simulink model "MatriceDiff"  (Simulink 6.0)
settings: Solver=ode45  StartTime=0  StopTime=17*t0  RelTol=1e-3
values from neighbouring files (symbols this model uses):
  b = S/Sm    (= 0.1)    [Constantes.m]    (also in ConstantesBck.m)
  beta = 0.95    [Constantes.m]    (also in ConstantesBck.m; ResCourV1.m = 1; ResCrV1.m = 1; ResEnerV1.m = 1)
  C = 1    [Constantes.m]    (also in ConstantesBck.m)
  gk = 36    [Constantes.m]    (also in ConstantesBck.m; sim_hh.m)
  gl = 0.3    [Constantes.m]    (also in ConstantesBck.m; sim_hh.m)
  gna = 120    [Constantes.m]    (also in ConstantesBck.m; sim_hh.m)
  h0 = 0.5961    [Constantes.m]    (also in ConstantesBck.m)
  m0 = 0.0529    [Constantes.m]    (also in ConstantesBck.m)
  mK = 0    [Constantes.m]    (also in ConstantesBck.m)
  mL = 0    [Constantes.m]    (also in ConstantesBck.m)
  mNa = 0    [Constantes.m]    (also in ConstantesBck.m)
  N = [6,8,5,5,7,1,2,6,9,1,1,9,4,8,8,7]    [Constantes.m]    (also in ConstantesBck.m; ImpedanceZtissus.m = 100; Ztissus.m = 100; charge.m = N(:,2))
  n0 = 0.3177    [Constantes.m]    (also in ConstantesBck.m)
  rapportIE = 10    [Constantes.m]
  Sm = 3.14e-2    (= 0.0314)    [Constantes.m]    (also in ConstantesBck.m = 0.000314)
  t0 = 2E-3    (= 0.002)    [Constantes.m]    (also in ConstantesBck.m = 0.001)
  Vk = -82    [Constantes.m]    (also in ConstantesBck.m)
  Vl = -59    [Constantes.m]    (also in ConstantesBck.m)
  Vna = 45    [Constantes.m]    (also in ConstantesBck.m)
  Vr = -70    [Constantes.m]    (also in ConstantesBck.m)
undefined symbols (not defined in the file or in its folder): ln
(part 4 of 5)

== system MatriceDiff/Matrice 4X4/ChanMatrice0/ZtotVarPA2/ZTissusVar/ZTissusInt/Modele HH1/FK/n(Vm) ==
  note: V
  note: alpha_*(1-n)
  note: beta_n*n
  note: n
  note: n
  Vm : Inport  Port=1  LatchInput=off
  (1-n) : Fcn  Expr=1-u
  Integrator1 : Integrator  InitialCondition=n0
  Product : Product
  Product1 : Product
  Sum1 : Sum  Inputs=+-
  V : Fcn  Expr=u-Vr
  alpha_n : Fcn  Expr=(0.01*(10-u))/(exp((10-u)/10)-1)
  beta_n : Fcn  Expr=0.125*exp(-u/80)
  n : Outport  InitialOutput=0
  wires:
  V/1 -> alpha_n/1, beta_n/1
  alpha_n/1 -> Product/2
  (1-n)/1 -> Product/1
  beta_n/1 -> Product1/1
  Product/1 -> Sum1/1
  Product1/1 -> Sum1/2
  Sum1/1 -> Integrator1/1
  Integrator1/1 -> (1-n)/1, Product1/2, n/1
  Vm/1 -> V/1

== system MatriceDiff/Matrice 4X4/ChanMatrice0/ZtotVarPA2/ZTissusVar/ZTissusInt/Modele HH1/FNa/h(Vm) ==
  note: h
  note: h
  note: beta_h*h
  note: alpha_h*(1-h)
  note: V
  Vm : Inport  Port=1  LatchInput=off
  (1-h) : Fcn  Expr=1-u
  Integrator1 : Integrator  InitialCondition=h0
  Product : Product
  Product1 : Product
  Sum1 : Sum  Inputs=+-
  V : Fcn  Expr=u-Vr
  alpha_h : Fcn  Expr=0.07*exp(-u/20)
  beta_h : Fcn  Expr=1/(exp((30-u)/10)+1)
  h : Outport  InitialOutput=0
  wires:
  Vm/1 -> V/1
  Integrator1/1 -> h/1, Product1/2, (1-h)/1
  Sum1/1 -> Integrator1/1
  Product1/1 -> Sum1/2
  Product/1 -> Sum1/1
  beta_h/1 -> Product1/1
  (1-h)/1 -> Product/1
  alpha_h/1 -> Product/2
  V/1 -> beta_h/1, alpha_h/1

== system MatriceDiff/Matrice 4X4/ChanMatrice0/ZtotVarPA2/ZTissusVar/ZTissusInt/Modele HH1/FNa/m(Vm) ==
  note: m
  note: m
  note: beta_m*m
  note: alpha_m*(1-m)
  note: V
  Vm : Inport  Port=1  LatchInput=off
  (1-m) : Fcn  Expr=1-u
  Integrator1 : Integrator  InitialCondition=m0
  Product : Product
  Product1 : Product
  Sum1 : Sum  Inputs=+-
  V : Fcn  Expr=u-Vr
  alpha_m : Fcn  Expr=(0.1*(25-u))/(exp((25-u)/10)-1)
  beta_m : Fcn  Expr=4*exp(-u/18)
  n : Outport  InitialOutput=0
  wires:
  Vm/1 -> V/1
  Integrator1/1 -> n/1, Product1/2, (1-m)/1
  Sum1/1 -> Integrator1/1
  Product1/1 -> Sum1/2
  Product/1 -> Sum1/1
  beta_m/1 -> Product1/1
  (1-m)/1 -> Product/1
  alpha_m/1 -> Product/2
  V/1 -> beta_m/1, alpha_m/1

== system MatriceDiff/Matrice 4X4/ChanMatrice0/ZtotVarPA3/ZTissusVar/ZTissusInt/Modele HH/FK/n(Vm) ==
  note: V
  note: alpha_*(1-n)
  note: beta_n*n
  note: n
  note: n
  Vm : Inport  Port=1  LatchInput=off
  (1-n) : Fcn  Expr=1-u
  Integrator1 : Integrator  InitialCondition=n0
  Product : Product
  Product1 : Product
  Sum1 : Sum  Inputs=+-
  V : Fcn  Expr=u-Vr
  alpha_n : Fcn  Expr=(0.01*(10-u))/(exp((10-u)/10)-1)
  beta_n : Fcn  Expr=0.125*exp(-u/80)
  n : Outport  InitialOutput=0
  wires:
  V/1 -> alpha_n/1, beta_n/1
  alpha_n/1 -> Product/2
  (1-n)/1 -> Product/1
  beta_n/1 -> Product1/1
  Product/1 -> Sum1/1
  Product1/1 -> Sum1/2
  Sum1/1 -> Integrator1/1
  Integrator1/1 -> (1-n)/1, Product1/2, n/1
  Vm/1 -> V/1

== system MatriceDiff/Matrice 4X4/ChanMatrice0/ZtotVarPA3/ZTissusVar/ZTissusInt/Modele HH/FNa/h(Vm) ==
  note: h
  note: h
  note: beta_h*h
  note: alpha_h*(1-h)
  note: V
  Vm : Inport  Port=1  LatchInput=off
  (1-h) : Fcn  Expr=1-u
  Integrator1 : Integrator  InitialCondition=h0
  Product : Product
  Product1 : Product
  Sum1 : Sum  Inputs=+-
  V : Fcn  Expr=u-Vr
  alpha_h : Fcn  Expr=0.07*exp(-u/20)
  beta_h : Fcn  Expr=1/(exp((30-u)/10)+1)
  h : Outport  InitialOutput=0
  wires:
  Vm/1 -> V/1
  Integrator1/1 -> h/1, Product1/2, (1-h)/1
  Sum1/1 -> Integrator1/1
  Product1/1 -> Sum1/2
  Product/1 -> Sum1/1
  beta_h/1 -> Product1/1
  (1-h)/1 -> Product/1
  alpha_h/1 -> Product/2
  V/1 -> beta_h/1, alpha_h/1

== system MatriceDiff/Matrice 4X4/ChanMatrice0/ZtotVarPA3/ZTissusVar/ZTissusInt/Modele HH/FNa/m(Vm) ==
  note: m
  note: m
  note: beta_m*m
  note: alpha_m*(1-m)
  note: V
  Vm : Inport  Port=1  LatchInput=off
  (1-m) : Fcn  Expr=1-u
  Integrator1 : Integrator  InitialCondition=m0
  Product : Product
  Product1 : Product
  Sum1 : Sum  Inputs=+-
  V : Fcn  Expr=u-Vr
  alpha_m : Fcn  Expr=(0.1*(25-u))/(exp((25-u)/10)-1)
  beta_m : Fcn  Expr=4*exp(-u/18)
  n : Outport  InitialOutput=0
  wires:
  Vm/1 -> V/1
  Integrator1/1 -> n/1, Product1/2, (1-m)/1
  Sum1/1 -> Integrator1/1
  Product1/1 -> Sum1/2
  Product/1 -> Sum1/1
  beta_m/1 -> Product1/1
  (1-m)/1 -> Product/1
  alpha_m/1 -> Product/2
  V/1 -> beta_m/1, alpha_m/1

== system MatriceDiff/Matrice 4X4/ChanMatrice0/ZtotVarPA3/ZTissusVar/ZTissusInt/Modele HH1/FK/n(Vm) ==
  note: V
  note: alpha_*(1-n)
  note: beta_n*n
  note: n
  note: n
  Vm : Inport  Port=1  LatchInput=off
  (1-n) : Fcn  Expr=1-u
  Integrator1 : Integrator  InitialCondition=n0
  Product : Product
  Product1 : Product
  Sum1 : Sum  Inputs=+-
  V : Fcn  Expr=u-Vr
  alpha_n : Fcn  Expr=(0.01*(10-u))/(exp((10-u)/10)-1)
  beta_n : Fcn  Expr=0.125*exp(-u/80)
  n : Outport  InitialOutput=0
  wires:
  V/1 -> alpha_n/1, beta_n/1
  alpha_n/1 -> Product/2
  (1-n)/1 -> Product/1
  beta_n/1 -> Product1/1
  Product/1 -> Sum1/1
  Product1/1 -> Sum1/2
  Sum1/1 -> Integrator1/1
  Integrator1/1 -> (1-n)/1, Product1/2, n/1
  Vm/1 -> V/1

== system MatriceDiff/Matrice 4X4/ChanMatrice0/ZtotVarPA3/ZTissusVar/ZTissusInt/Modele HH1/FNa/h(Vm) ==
  note: h
  note: h
  note: beta_h*h
  note: alpha_h*(1-h)
  note: V
  Vm : Inport  Port=1  LatchInput=off
  (1-h) : Fcn  Expr=1-u
  Integrator1 : Integrator  InitialCondition=h0
  Product : Product
  Product1 : Product
  Sum1 : Sum  Inputs=+-
  V : Fcn  Expr=u-Vr
  alpha_h : Fcn  Expr=0.07*exp(-u/20)
  beta_h : Fcn  Expr=1/(exp((30-u)/10)+1)
  h : Outport  InitialOutput=0
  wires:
  Vm/1 -> V/1
  Integrator1/1 -> h/1, Product1/2, (1-h)/1
  Sum1/1 -> Integrator1/1
  Product1/1 -> Sum1/2
  Product/1 -> Sum1/1
  beta_h/1 -> Product1/1
  (1-h)/1 -> Product/1
  alpha_h/1 -> Product/2
  V/1 -> beta_h/1, alpha_h/1

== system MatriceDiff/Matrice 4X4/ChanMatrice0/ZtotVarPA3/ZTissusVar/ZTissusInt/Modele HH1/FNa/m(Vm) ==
  note: m
  note: m
  note: beta_m*m
  note: alpha_m*(1-m)
  note: V
  Vm : Inport  Port=1  LatchInput=off
  (1-m) : Fcn  Expr=1-u
  Integrator1 : Integrator  InitialCondition=m0
  Product : Product
  Product1 : Product
  Sum1 : Sum  Inputs=+-
  V : Fcn  Expr=u-Vr
  alpha_m : Fcn  Expr=(0.1*(25-u))/(exp((25-u)/10)-1)
  beta_m : Fcn  Expr=4*exp(-u/18)
  n : Outport  InitialOutput=0
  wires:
  Vm/1 -> V/1
  Integrator1/1 -> n/1, Product1/2, (1-m)/1
  Sum1/1 -> Integrator1/1
  Product1/1 -> Sum1/2
  Product/1 -> Sum1/1
  beta_m/1 -> Product1/1
  (1-m)/1 -> Product/1
  alpha_m/1 -> Product/2
  V/1 -> beta_m/1, alpha_m/1

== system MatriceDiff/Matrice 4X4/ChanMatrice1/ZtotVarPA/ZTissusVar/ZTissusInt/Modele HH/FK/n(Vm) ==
  note: V
  note: alpha_*(1-n)
  note: beta_n*n
  note: n
  note: n
  Vm : Inport  Port=1  LatchInput=off
  (1-n) : Fcn  Expr=1-u
  Integrator1 : Integrator  InitialCondition=n0
  Product : Product
  Product1 : Product
  Sum1 : Sum  Inputs=+-
  V : Fcn  Expr=u-Vr
  alpha_n : Fcn  Expr=(0.01*(10-u))/(exp((10-u)/10)-1)
  beta_n : Fcn  Expr=0.125*exp(-u/80)
  n : Outport  InitialOutput=0
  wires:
  V/1 -> alpha_n/1, beta_n/1
  alpha_n/1 -> Product/2
  (1-n)/1 -> Product/1
  beta_n/1 -> Product1/1
  Product/1 -> Sum1/1
  Product1/1 -> Sum1/2
  Sum1/1 -> Integrator1/1
  Integrator1/1 -> (1-n)/1, Product1/2, n/1
  Vm/1 -> V/1

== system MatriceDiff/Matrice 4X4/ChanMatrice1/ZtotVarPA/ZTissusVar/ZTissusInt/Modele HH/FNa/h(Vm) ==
  note: h
  note: h
  note: beta_h*h
  note: alpha_h*(1-h)
  note: V
  Vm : Inport  Port=1  LatchInput=off
  (1-h) : Fcn  Expr=1-u
  Integrator1 : Integrator  InitialCondition=h0
  Product : Product
  Product1 : Product
  Sum1 : Sum  Inputs=+-
  V : Fcn  Expr=u-Vr
  alpha_h : Fcn  Expr=0.07*exp(-u/20)
  beta_h : Fcn  Expr=1/(exp((30-u)/10)+1)
  h : Outport  InitialOutput=0
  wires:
  Vm/1 -> V/1
  Integrator1/1 -> h/1, Product1/2, (1-h)/1
  Sum1/1 -> Integrator1/1
  Product1/1 -> Sum1/2
  Product/1 -> Sum1/1
  beta_h/1 -> Product1/1
  (1-h)/1 -> Product/1
  alpha_h/1 -> Product/2
  V/1 -> beta_h/1, alpha_h/1

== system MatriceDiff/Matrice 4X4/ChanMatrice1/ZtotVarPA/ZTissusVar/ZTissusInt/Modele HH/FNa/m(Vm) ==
  note: m
  note: m
  note: beta_m*m
  note: alpha_m*(1-m)
  note: V
  Vm : Inport  Port=1  LatchInput=off
  (1-m) : Fcn  Expr=1-u
  Integrator1 : Integrator  InitialCondition=m0
  Product : Product
  Product1 : Product
  Sum1 : Sum  Inputs=+-
  V : Fcn  Expr=u-Vr
  alpha_m : Fcn  Expr=(0.1*(25-u))/(exp((25-u)/10)-1)
  beta_m : Fcn  Expr=4*exp(-u/18)
  n : Outport  InitialOutput=0
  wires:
  Vm/1 -> V/1
  Integrator1/1 -> n/1, Product1/2, (1-m)/1
  Sum1/1 -> Integrator1/1
  Product1/1 -> Sum1/2
  Product/1 -> Sum1/1
  beta_m/1 -> Product1/1
  (1-m)/1 -> Product/1
  alpha_m/1 -> Product/2
  V/1 -> beta_m/1, alpha_m/1

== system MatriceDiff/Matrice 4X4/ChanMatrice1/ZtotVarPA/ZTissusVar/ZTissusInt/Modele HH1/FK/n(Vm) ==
  note: V
  note: alpha_*(1-n)
  note: beta_n*n
  note: n
  note: n
  Vm : Inport  Port=1  LatchInput=off
  (1-n) : Fcn  Expr=1-u
  Integrator1 : Integrator  InitialCondition=n0
  Product : Product
  Product1 : Product
  Sum1 : Sum  Inputs=+-
  V : Fcn  Expr=u-Vr
  alpha_n : Fcn  Expr=(0.01*(10-u))/(exp((10-u)/10)-1)
  beta_n : Fcn  Expr=0.125*exp(-u/80)
  n : Outport  InitialOutput=0
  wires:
  V/1 -> alpha_n/1, beta_n/1
  alpha_n/1 -> Product/2
  (1-n)/1 -> Product/1
  beta_n/1 -> Product1/1
  Product/1 -> Sum1/1
  Product1/1 -> Sum1/2
  Sum1/1 -> Integrator1/1
  Integrator1/1 -> (1-n)/1, Product1/2, n/1
  Vm/1 -> V/1

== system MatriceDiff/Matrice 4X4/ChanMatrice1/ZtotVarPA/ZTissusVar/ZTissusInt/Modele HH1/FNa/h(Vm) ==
  note: h
  note: h
  note: beta_h*h
  note: alpha_h*(1-h)
  note: V
  Vm : Inport  Port=1  LatchInput=off
  (1-h) : Fcn  Expr=1-u
  Integrator1 : Integrator  InitialCondition=h0
  Product : Product
  Product1 : Product
  Sum1 : Sum  Inputs=+-
  V : Fcn  Expr=u-Vr
  alpha_h : Fcn  Expr=0.07*exp(-u/20)
  beta_h : Fcn  Expr=1/(exp((30-u)/10)+1)
  h : Outport  InitialOutput=0
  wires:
  Vm/1 -> V/1
  Integrator1/1 -> h/1, Product1/2, (1-h)/1
  Sum1/1 -> Integrator1/1
  Product1/1 -> Sum1/2
  Product/1 -> Sum1/1
  beta_h/1 -> Product1/1
  (1-h)/1 -> Product/1
  alpha_h/1 -> Product/2
  V/1 -> beta_h/1, alpha_h/1

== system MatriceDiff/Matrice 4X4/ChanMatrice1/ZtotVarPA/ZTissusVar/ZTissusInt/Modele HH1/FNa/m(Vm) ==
  note: m
  note: m
  note: beta_m*m
  note: alpha_m*(1-m)
  note: V
  Vm : Inport  Port=1  LatchInput=off
  (1-m) : Fcn  Expr=1-u
  Integrator1 : Integrator  InitialCondition=m0
  Product : Product
  Product1 : Product
  Sum1 : Sum  Inputs=+-
  V : Fcn  Expr=u-Vr
  alpha_m : Fcn  Expr=(0.1*(25-u))/(exp((25-u)/10)-1)
  beta_m : Fcn  Expr=4*exp(-u/18)
  n : Outport  InitialOutput=0
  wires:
  Vm/1 -> V/1
  Integrator1/1 -> n/1, Product1/2, (1-m)/1
  Sum1/1 -> Integrator1/1
  Product1/1 -> Sum1/2
  Product/1 -> Sum1/1
  beta_m/1 -> Product1/1
  (1-m)/1 -> Product/1
  alpha_m/1 -> Product/2
  V/1 -> beta_m/1, alpha_m/1

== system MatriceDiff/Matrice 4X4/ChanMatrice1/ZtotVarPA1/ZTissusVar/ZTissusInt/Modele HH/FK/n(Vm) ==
  note: V
  note: alpha_*(1-n)
  note: beta_n*n
  note: n
  note: n
  Vm : Inport  Port=1  LatchInput=off
  (1-n) : Fcn  Expr=1-u
  Integrator1 : Integrator  InitialCondition=n0
  Product : Product
  Product1 : Product
  Sum1 : Sum  Inputs=+-
  V : Fcn  Expr=u-Vr
  alpha_n : Fcn  Expr=(0.01*(10-u))/(exp((10-u)/10)-1)
  beta_n : Fcn  Expr=0.125*exp(-u/80)
  n : Outport  InitialOutput=0
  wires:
  V/1 -> alpha_n/1, beta_n/1
  alpha_n/1 -> Product/2
  (1-n)/1 -> Product/1
  beta_n/1 -> Product1/1
  Product/1 -> Sum1/1
  Product1/1 -> Sum1/2
  Sum1/1 -> Integrator1/1
  Integrator1/1 -> (1-n)/1, Product1/2, n/1
  Vm/1 -> V/1

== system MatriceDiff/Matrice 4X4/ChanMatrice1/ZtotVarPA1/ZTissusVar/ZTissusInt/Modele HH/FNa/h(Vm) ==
  note: h
  note: h
  note: beta_h*h
  note: alpha_h*(1-h)
  note: V
  Vm : Inport  Port=1  LatchInput=off
  (1-h) : Fcn  Expr=1-u
  Integrator1 : Integrator  InitialCondition=h0
  Product : Product
  Product1 : Product
  Sum1 : Sum  Inputs=+-
  V : Fcn  Expr=u-Vr
  alpha_h : Fcn  Expr=0.07*exp(-u/20)
  beta_h : Fcn  Expr=1/(exp((30-u)/10)+1)
  h : Outport  InitialOutput=0
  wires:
  Vm/1 -> V/1
  Integrator1/1 -> h/1, Product1/2, (1-h)/1
  Sum1/1 -> Integrator1/1
  Product1/1 -> Sum1/2
  Product/1 -> Sum1/1
  beta_h/1 -> Product1/1
  (1-h)/1 -> Product/1
  alpha_h/1 -> Product/2
  V/1 -> beta_h/1, alpha_h/1

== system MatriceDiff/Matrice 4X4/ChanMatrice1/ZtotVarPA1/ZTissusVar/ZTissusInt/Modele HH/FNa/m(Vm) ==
  note: m
  note: m
  note: beta_m*m
  note: alpha_m*(1-m)
  note: V
  Vm : Inport  Port=1  LatchInput=off
  (1-m) : Fcn  Expr=1-u
  Integrator1 : Integrator  InitialCondition=m0
  Product : Product
  Product1 : Product
  Sum1 : Sum  Inputs=+-
  V : Fcn  Expr=u-Vr
  alpha_m : Fcn  Expr=(0.1*(25-u))/(exp((25-u)/10)-1)
  beta_m : Fcn  Expr=4*exp(-u/18)
  n : Outport  InitialOutput=0
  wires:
  Vm/1 -> V/1
  Integrator1/1 -> n/1, Product1/2, (1-m)/1
  Sum1/1 -> Integrator1/1
  Product1/1 -> Sum1/2
  Product/1 -> Sum1/1
  beta_m/1 -> Product1/1
  (1-m)/1 -> Product/1
  alpha_m/1 -> Product/2
  V/1 -> beta_m/1, alpha_m/1

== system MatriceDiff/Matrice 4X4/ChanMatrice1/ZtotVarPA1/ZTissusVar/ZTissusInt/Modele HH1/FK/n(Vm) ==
  note: V
  note: alpha_*(1-n)
  note: beta_n*n
  note: n
  note: n
  Vm : Inport  Port=1  LatchInput=off
  (1-n) : Fcn  Expr=1-u
  Integrator1 : Integrator  InitialCondition=n0
  Product : Product
  Product1 : Product
  Sum1 : Sum  Inputs=+-
  V : Fcn  Expr=u-Vr
  alpha_n : Fcn  Expr=(0.01*(10-u))/(exp((10-u)/10)-1)
  beta_n : Fcn  Expr=0.125*exp(-u/80)
  n : Outport  InitialOutput=0
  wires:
  V/1 -> alpha_n/1, beta_n/1
  alpha_n/1 -> Product/2
  (1-n)/1 -> Product/1
  beta_n/1 -> Product1/1
  Product/1 -> Sum1/1
  Product1/1 -> Sum1/2
  Sum1/1 -> Integrator1/1
  Integrator1/1 -> (1-n)/1, Product1/2, n/1
  Vm/1 -> V/1

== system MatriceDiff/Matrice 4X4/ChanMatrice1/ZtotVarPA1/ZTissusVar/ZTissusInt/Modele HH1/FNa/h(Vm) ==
  note: h
  note: h
  note: beta_h*h
  note: alpha_h*(1-h)
  note: V
  Vm : Inport  Port=1  LatchInput=off
  (1-h) : Fcn  Expr=1-u
  Integrator1 : Integrator  InitialCondition=h0
  Product : Product
  Product1 : Product
  Sum1 : Sum  Inputs=+-
  V : Fcn  Expr=u-Vr
  alpha_h : Fcn  Expr=0.07*exp(-u/20)
  beta_h : Fcn  Expr=1/(exp((30-u)/10)+1)
  h : Outport  InitialOutput=0
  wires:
  Vm/1 -> V/1
  Integrator1/1 -> h/1, Product1/2, (1-h)/1
  Sum1/1 -> Integrator1/1
  Product1/1 -> Sum1/2
  Product/1 -> Sum1/1
  beta_h/1 -> Product1/1
  (1-h)/1 -> Product/1
  alpha_h/1 -> Product/2
  V/1 -> beta_h/1, alpha_h/1

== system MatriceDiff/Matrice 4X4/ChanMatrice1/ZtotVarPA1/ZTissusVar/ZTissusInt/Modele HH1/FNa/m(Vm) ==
  note: m
  note: m
  note: beta_m*m
  note: alpha_m*(1-m)
  note: V
  Vm : Inport  Port=1  LatchInput=off
  (1-m) : Fcn  Expr=1-u
  Integrator1 : Integrator  InitialCondition=m0
  Product : Product
  Product1 : Product
  Sum1 : Sum  Inputs=+-
  V : Fcn  Expr=u-Vr
  alpha_m : Fcn  Expr=(0.1*(25-u))/(exp((25-u)/10)-1)
  beta_m : Fcn  Expr=4*exp(-u/18)
  n : Outport  InitialOutput=0
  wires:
  Vm/1 -> V/1
  Integrator1/1 -> n/1, Product1/2, (1-m)/1
  Sum1/1 -> Integrator1/1
  Product1/1 -> Sum1/2
  Product/1 -> Sum1/1
  beta_m/1 -> Product1/1
  (1-m)/1 -> Product/1
  alpha_m/1 -> Product/2
  V/1 -> beta_m/1, alpha_m/1

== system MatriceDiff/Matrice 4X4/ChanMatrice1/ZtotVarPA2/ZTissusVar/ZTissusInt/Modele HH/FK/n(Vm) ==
  note: V
  note: alpha_*(1-n)
  note: beta_n*n
  note: n
  note: n
  Vm : Inport  Port=1  LatchInput=off
  (1-n) : Fcn  Expr=1-u
  Integrator1 : Integrator  InitialCondition=n0
  Product : Product
  Product1 : Product
  Sum1 : Sum  Inputs=+-
  V : Fcn  Expr=u-Vr
  alpha_n : Fcn  Expr=(0.01*(10-u))/(exp((10-u)/10)-1)
  beta_n : Fcn  Expr=0.125*exp(-u/80)
  n : Outport  InitialOutput=0
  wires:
  V/1 -> alpha_n/1, beta_n/1
  alpha_n/1 -> Product/2
  (1-n)/1 -> Product/1
  beta_n/1 -> Product1/1
  Product/1 -> Sum1/1
  Product1/1 -> Sum1/2
  Sum1/1 -> Integrator1/1
  Integrator1/1 -> (1-n)/1, Product1/2, n/1
  Vm/1 -> V/1

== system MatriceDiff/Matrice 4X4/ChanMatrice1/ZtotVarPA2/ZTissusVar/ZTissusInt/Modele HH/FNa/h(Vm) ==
  note: h
  note: h
  note: beta_h*h
  note: alpha_h*(1-h)
  note: V
  Vm : Inport  Port=1  LatchInput=off
  (1-h) : Fcn  Expr=1-u
  Integrator1 : Integrator  InitialCondition=h0
  Product : Product
  Product1 : Product
  Sum1 : Sum  Inputs=+-
  V : Fcn  Expr=u-Vr
  alpha_h : Fcn  Expr=0.07*exp(-u/20)
  beta_h : Fcn  Expr=1/(exp((30-u)/10)+1)
  h : Outport  InitialOutput=0
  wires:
  Vm/1 -> V/1
  Integrator1/1 -> h/1, Product1/2, (1-h)/1
  Sum1/1 -> Integrator1/1
  Product1/1 -> Sum1/2
  Product/1 -> Sum1/1
  beta_h/1 -> Product1/1
  (1-h)/1 -> Product/1
  alpha_h/1 -> Product/2
  V/1 -> beta_h/1, alpha_h/1

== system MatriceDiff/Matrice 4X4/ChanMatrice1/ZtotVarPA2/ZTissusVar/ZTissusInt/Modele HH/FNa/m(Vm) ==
  note: m
  note: m
  note: beta_m*m
  note: alpha_m*(1-m)
  note: V
  Vm : Inport  Port=1  LatchInput=off
  (1-m) : Fcn  Expr=1-u
  Integrator1 : Integrator  InitialCondition=m0
  Product : Product
  Product1 : Product
  Sum1 : Sum  Inputs=+-
  V : Fcn  Expr=u-Vr
  alpha_m : Fcn  Expr=(0.1*(25-u))/(exp((25-u)/10)-1)
  beta_m : Fcn  Expr=4*exp(-u/18)
  n : Outport  InitialOutput=0
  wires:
  Vm/1 -> V/1
  Integrator1/1 -> n/1, Product1/2, (1-m)/1
  Sum1/1 -> Integrator1/1
  Product1/1 -> Sum1/2
  Product/1 -> Sum1/1
  beta_m/1 -> Product1/1
  (1-m)/1 -> Product/1
  alpha_m/1 -> Product/2
  V/1 -> beta_m/1, alpha_m/1

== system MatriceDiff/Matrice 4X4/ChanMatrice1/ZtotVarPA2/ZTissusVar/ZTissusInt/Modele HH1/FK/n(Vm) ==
  note: V
  note: alpha_*(1-n)
  note: beta_n*n
  note: n
  note: n
  Vm : Inport  Port=1  LatchInput=off
  (1-n) : Fcn  Expr=1-u
  Integrator1 : Integrator  InitialCondition=n0
  Product : Product
  Product1 : Product
  Sum1 : Sum  Inputs=+-
  V : Fcn  Expr=u-Vr
  alpha_n : Fcn  Expr=(0.01*(10-u))/(exp((10-u)/10)-1)
  beta_n : Fcn  Expr=0.125*exp(-u/80)
  n : Outport  InitialOutput=0
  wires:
  V/1 -> alpha_n/1, beta_n/1
  alpha_n/1 -> Product/2
  (1-n)/1 -> Product/1
  beta_n/1 -> Product1/1
  Product/1 -> Sum1/1
  Product1/1 -> Sum1/2
  Sum1/1 -> Integrator1/1
  Integrator1/1 -> (1-n)/1, Product1/2, n/1
  Vm/1 -> V/1

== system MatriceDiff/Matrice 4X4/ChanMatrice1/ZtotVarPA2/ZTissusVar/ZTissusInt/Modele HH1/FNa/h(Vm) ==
  note: h
  note: h
  note: beta_h*h
  note: alpha_h*(1-h)
  note: V
  Vm : Inport  Port=1  LatchInput=off
  (1-h) : Fcn  Expr=1-u
  Integrator1 : Integrator  InitialCondition=h0
  Product : Product
  Product1 : Product
  Sum1 : Sum  Inputs=+-
  V : Fcn  Expr=u-Vr
  alpha_h : Fcn  Expr=0.07*exp(-u/20)
  beta_h : Fcn  Expr=1/(exp((30-u)/10)+1)
  h : Outport  InitialOutput=0
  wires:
  Vm/1 -> V/1
  Integrator1/1 -> h/1, Product1/2, (1-h)/1
  Sum1/1 -> Integrator1/1
  Product1/1 -> Sum1/2
  Product/1 -> Sum1/1
  beta_h/1 -> Product1/1
  (1-h)/1 -> Product/1
  alpha_h/1 -> Product/2
  V/1 -> beta_h/1, alpha_h/1

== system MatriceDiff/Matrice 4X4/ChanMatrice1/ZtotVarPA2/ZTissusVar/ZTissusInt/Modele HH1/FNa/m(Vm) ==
  note: m
  note: m
  note: beta_m*m
  note: alpha_m*(1-m)
  note: V
  Vm : Inport  Port=1  LatchInput=off
  (1-m) : Fcn  Expr=1-u
  Integrator1 : Integrator  InitialCondition=m0
  Product : Product
  Product1 : Product
  Sum1 : Sum  Inputs=+-
  V : Fcn  Expr=u-Vr
  alpha_m : Fcn  Expr=(0.1*(25-u))/(exp((25-u)/10)-1)
  beta_m : Fcn  Expr=4*exp(-u/18)
  n : Outport  InitialOutput=0
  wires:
  Vm/1 -> V/1
  Integrator1/1 -> n/1, Product1/2, (1-m)/1
  Sum1/1 -> Integrator1/1
  Product1/1 -> Sum1/2
  Product/1 -> Sum1/1
  beta_m/1 -> Product1/1
  (1-m)/1 -> Product/1
  alpha_m/1 -> Product/2
  V/1 -> beta_m/1, alpha_m/1

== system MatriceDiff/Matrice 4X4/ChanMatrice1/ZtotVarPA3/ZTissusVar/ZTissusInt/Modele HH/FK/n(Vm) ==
  note: V
  note: alpha_*(1-n)
  note: beta_n*n
  note: n
  note: n
  Vm : Inport  Port=1  LatchInput=off
  (1-n) : Fcn  Expr=1-u
  Integrator1 : Integrator  InitialCondition=n0
  Product : Product
  Product1 : Product
  Sum1 : Sum  Inputs=+-
  V : Fcn  Expr=u-Vr
  alpha_n : Fcn  Expr=(0.01*(10-u))/(exp((10-u)/10)-1)
  beta_n : Fcn  Expr=0.125*exp(-u/80)
  n : Outport  InitialOutput=0
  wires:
  V/1 -> alpha_n/1, beta_n/1
  alpha_n/1 -> Product/2
  (1-n)/1 -> Product/1
  beta_n/1 -> Product1/1
  Product/1 -> Sum1/1
  Product1/1 -> Sum1/2
  Sum1/1 -> Integrator1/1
  Integrator1/1 -> (1-n)/1, Product1/2, n/1
  Vm/1 -> V/1

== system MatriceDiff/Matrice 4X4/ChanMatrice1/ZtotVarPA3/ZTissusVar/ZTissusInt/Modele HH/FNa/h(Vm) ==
  note: h
  note: h
  note: beta_h*h
  note: alpha_h*(1-h)
  note: V
  Vm : Inport  Port=1  LatchInput=off
  (1-h) : Fcn  Expr=1-u
  Integrator1 : Integrator  InitialCondition=h0
  Product : Product
  Product1 : Product
  Sum1 : Sum  Inputs=+-
  V : Fcn  Expr=u-Vr
  alpha_h : Fcn  Expr=0.07*exp(-u/20)
  beta_h : Fcn  Expr=1/(exp((30-u)/10)+1)
  h : Outport  InitialOutput=0
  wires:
  Vm/1 -> V/1
  Integrator1/1 -> h/1, Product1/2, (1-h)/1
  Sum1/1 -> Integrator1/1
  Product1/1 -> Sum1/2
  Product/1 -> Sum1/1
  beta_h/1 -> Product1/1
  (1-h)/1 -> Product/1
  alpha_h/1 -> Product/2
  V/1 -> beta_h/1, alpha_h/1

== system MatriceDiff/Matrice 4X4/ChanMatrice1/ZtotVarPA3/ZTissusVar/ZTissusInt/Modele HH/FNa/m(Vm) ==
  note: m
  note: m
  note: beta_m*m
  note: alpha_m*(1-m)
  note: V
  Vm : Inport  Port=1  LatchInput=off
  (1-m) : Fcn  Expr=1-u
  Integrator1 : Integrator  InitialCondition=m0
  Product : Product
  Product1 : Product
  Sum1 : Sum  Inputs=+-
  V : Fcn  Expr=u-Vr
  alpha_m : Fcn  Expr=(0.1*(25-u))/(exp((25-u)/10)-1)
  beta_m : Fcn  Expr=4*exp(-u/18)
  n : Outport  InitialOutput=0
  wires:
  Vm/1 -> V/1
  Integrator1/1 -> n/1, Product1/2, (1-m)/1
  Sum1/1 -> Integrator1/1
  Product1/1 -> Sum1/2
  Product/1 -> Sum1/1
  beta_m/1 -> Product1/1
  (1-m)/1 -> Product/1
  alpha_m/1 -> Product/2
  V/1 -> beta_m/1, alpha_m/1

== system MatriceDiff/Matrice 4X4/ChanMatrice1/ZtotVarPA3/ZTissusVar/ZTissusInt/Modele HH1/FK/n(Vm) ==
  note: V
  note: alpha_*(1-n)
  note: beta_n*n
  note: n
  note: n
  Vm : Inport  Port=1  LatchInput=off
  (1-n) : Fcn  Expr=1-u
  Integrator1 : Integrator  InitialCondition=n0
  Product : Product
  Product1 : Product
  Sum1 : Sum  Inputs=+-
  V : Fcn  Expr=u-Vr
  alpha_n : Fcn  Expr=(0.01*(10-u))/(exp((10-u)/10)-1)
  beta_n : Fcn  Expr=0.125*exp(-u/80)
  n : Outport  InitialOutput=0
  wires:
  V/1 -> alpha_n/1, beta_n/1
  alpha_n/1 -> Product/2
  (1-n)/1 -> Product/1
  beta_n/1 -> Product1/1
  Product/1 -> Sum1/1
  Product1/1 -> Sum1/2
  Sum1/1 -> Integrator1/1
  Integrator1/1 -> (1-n)/1, Product1/2, n/1
  Vm/1 -> V/1

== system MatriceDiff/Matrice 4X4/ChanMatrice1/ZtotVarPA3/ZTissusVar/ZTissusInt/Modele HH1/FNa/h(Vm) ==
  note: h
  note: h
  note: beta_h*h
  note: alpha_h*(1-h)
  note: V
  Vm : Inport  Port=1  LatchInput=off
  (1-h) : Fcn  Expr=1-u
  Integrator1 : Integrator  InitialCondition=h0
  Product : Product
  Product1 : Product
  Sum1 : Sum  Inputs=+-
  V : Fcn  Expr=u-Vr
  alpha_h : Fcn  Expr=0.07*exp(-u/20)
  beta_h : Fcn  Expr=1/(exp((30-u)/10)+1)
  h : Outport  InitialOutput=0
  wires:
  Vm/1 -> V/1
  Integrator1/1 -> h/1, Product1/2, (1-h)/1
  Sum1/1 -> Integrator1/1
  Product1/1 -> Sum1/2
  Product/1 -> Sum1/1
  beta_h/1 -> Product1/1
  (1-h)/1 -> Product/1
  alpha_h/1 -> Product/2
  V/1 -> beta_h/1, alpha_h/1

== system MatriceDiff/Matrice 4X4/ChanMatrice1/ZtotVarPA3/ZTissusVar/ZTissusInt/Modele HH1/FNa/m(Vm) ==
  note: m
  note: m
  note: beta_m*m
  note: alpha_m*(1-m)
  note: V
  Vm : Inport  Port=1  LatchInput=off
  (1-m) : Fcn  Expr=1-u
  Integrator1 : Integrator  InitialCondition=m0
  Product : Product
  Product1 : Product
  Sum1 : Sum  Inputs=+-
  V : Fcn  Expr=u-Vr
  alpha_m : Fcn  Expr=(0.1*(25-u))/(exp((25-u)/10)-1)
  beta_m : Fcn  Expr=4*exp(-u/18)
  n : Outport  InitialOutput=0
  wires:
  Vm/1 -> V/1
  Integrator1/1 -> n/1, Product1/2, (1-m)/1
  Sum1/1 -> Integrator1/1
  Product1/1 -> Sum1/2
  Product/1 -> Sum1/1
  beta_m/1 -> Product1/1
  (1-m)/1 -> Product/1
  alpha_m/1 -> Product/2
  V/1 -> beta_m/1, alpha_m/1

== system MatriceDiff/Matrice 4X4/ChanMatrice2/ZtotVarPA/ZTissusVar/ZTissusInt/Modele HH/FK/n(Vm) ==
  note: V
  note: alpha_*(1-n)
  note: beta_n*n
  note: n
  note: n
  Vm : Inport  Port=1  LatchInput=off
  (1-n) : Fcn  Expr=1-u
  Integrator1 : Integrator  InitialCondition=n0
  Product : Product
  Product1 : Product
  Sum1 : Sum  Inputs=+-
  V : Fcn  Expr=u-Vr
  alpha_n : Fcn  Expr=(0.01*(10-u))/(exp((10-u)/10)-1)
  beta_n : Fcn  Expr=0.125*exp(-u/80)
  n : Outport  InitialOutput=0
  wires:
  V/1 -> alpha_n/1, beta_n/1
  alpha_n/1 -> Product/2
  (1-n)/1 -> Product/1
  beta_n/1 -> Product1/1
  Product/1 -> Sum1/1
  Product1/1 -> Sum1/2
  Sum1/1 -> Integrator1/1
  Integrator1/1 -> (1-n)/1, Product1/2, n/1
  Vm/1 -> V/1

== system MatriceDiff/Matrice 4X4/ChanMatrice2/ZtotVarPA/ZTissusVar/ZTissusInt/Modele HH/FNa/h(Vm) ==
  note: h
  note: h
  note: beta_h*h
  note: alpha_h*(1-h)
  note: V
  Vm : Inport  Port=1  LatchInput=off
  (1-h) : Fcn  Expr=1-u
  Integrator1 : Integrator  InitialCondition=h0
  Product : Product
  Product1 : Product
  Sum1 : Sum  Inputs=+-
  V : Fcn  Expr=u-Vr
  alpha_h : Fcn  Expr=0.07*exp(-u/20)
  beta_h : Fcn  Expr=1/(exp((30-u)/10)+1)
  h : Outport  InitialOutput=0
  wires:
  Vm/1 -> V/1
  Integrator1/1 -> h/1, Product1/2, (1-h)/1
  Sum1/1 -> Integrator1/1
  Product1/1 -> Sum1/2
  Product/1 -> Sum1/1
  beta_h/1 -> Product1/1
  (1-h)/1 -> Product/1
  alpha_h/1 -> Product/2
  V/1 -> beta_h/1, alpha_h/1

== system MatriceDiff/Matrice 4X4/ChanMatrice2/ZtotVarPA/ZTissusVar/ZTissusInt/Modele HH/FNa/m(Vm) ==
  note: m
  note: m
  note: beta_m*m
  note: alpha_m*(1-m)
  note: V
  Vm : Inport  Port=1  LatchInput=off
  (1-m) : Fcn  Expr=1-u
  Integrator1 : Integrator  InitialCondition=m0
  Product : Product
  Product1 : Product
  Sum1 : Sum  Inputs=+-
  V : Fcn  Expr=u-Vr
  alpha_m : Fcn  Expr=(0.1*(25-u))/(exp((25-u)/10)-1)
  beta_m : Fcn  Expr=4*exp(-u/18)
  n : Outport  InitialOutput=0
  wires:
  Vm/1 -> V/1
  Integrator1/1 -> n/1, Product1/2, (1-m)/1
  Sum1/1 -> Integrator1/1
  Product1/1 -> Sum1/2
  Product/1 -> Sum1/1
  beta_m/1 -> Product1/1
  (1-m)/1 -> Product/1
  alpha_m/1 -> Product/2
  V/1 -> beta_m/1, alpha_m/1

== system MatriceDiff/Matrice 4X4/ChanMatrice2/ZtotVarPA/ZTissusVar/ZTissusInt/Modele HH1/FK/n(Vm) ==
  note: V
  note: alpha_*(1-n)
  note: beta_n*n
  note: n
  note: n
  Vm : Inport  Port=1  LatchInput=off
  (1-n) : Fcn  Expr=1-u
  Integrator1 : Integrator  InitialCondition=n0
  Product : Product
  Product1 : Product
  Sum1 : Sum  Inputs=+-
  V : Fcn  Expr=u-Vr
  alpha_n : Fcn  Expr=(0.01*(10-u))/(exp((10-u)/10)-1)
  beta_n : Fcn  Expr=0.125*exp(-u/80)
  n : Outport  InitialOutput=0
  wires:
  V/1 -> alpha_n/1, beta_n/1
  alpha_n/1 -> Product/2
  (1-n)/1 -> Product/1
  beta_n/1 -> Product1/1
  Product/1 -> Sum1/1
  Product1/1 -> Sum1/2
  Sum1/1 -> Integrator1/1
  Integrator1/1 -> (1-n)/1, Product1/2, n/1
  Vm/1 -> V/1

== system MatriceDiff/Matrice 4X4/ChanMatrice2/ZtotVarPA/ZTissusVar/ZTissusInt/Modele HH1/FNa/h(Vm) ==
  note: h
  note: h
  note: beta_h*h
  note: alpha_h*(1-h)
  note: V
  Vm : Inport  Port=1  LatchInput=off
  (1-h) : Fcn  Expr=1-u
  Integrator1 : Integrator  InitialCondition=h0
  Product : Product
  Product1 : Product
  Sum1 : Sum  Inputs=+-
  V : Fcn  Expr=u-Vr
  alpha_h : Fcn  Expr=0.07*exp(-u/20)
  beta_h : Fcn  Expr=1/(exp((30-u)/10)+1)
  h : Outport  InitialOutput=0
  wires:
  Vm/1 -> V/1
  Integrator1/1 -> h/1, Product1/2, (1-h)/1
  Sum1/1 -> Integrator1/1
  Product1/1 -> Sum1/2
  Product/1 -> Sum1/1
  beta_h/1 -> Product1/1
  (1-h)/1 -> Product/1
  alpha_h/1 -> Product/2
  V/1 -> beta_h/1, alpha_h/1

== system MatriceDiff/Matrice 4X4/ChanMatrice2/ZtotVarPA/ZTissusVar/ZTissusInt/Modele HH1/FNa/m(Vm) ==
  note: m
  note: m
  note: beta_m*m
  note: alpha_m*(1-m)
  note: V
  Vm : Inport  Port=1  LatchInput=off
  (1-m) : Fcn  Expr=1-u
  Integrator1 : Integrator  InitialCondition=m0
  Product : Product
  Product1 : Product
  Sum1 : Sum  Inputs=+-
  V : Fcn  Expr=u-Vr
  alpha_m : Fcn  Expr=(0.1*(25-u))/(exp((25-u)/10)-1)
  beta_m : Fcn  Expr=4*exp(-u/18)
  n : Outport  InitialOutput=0
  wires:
  Vm/1 -> V/1
  Integrator1/1 -> n/1, Product1/2, (1-m)/1
  Sum1/1 -> Integrator1/1
  Product1/1 -> Sum1/2
  Product/1 -> Sum1/1
  beta_m/1 -> Product1/1
  (1-m)/1 -> Product/1
  alpha_m/1 -> Product/2
  V/1 -> beta_m/1, alpha_m/1

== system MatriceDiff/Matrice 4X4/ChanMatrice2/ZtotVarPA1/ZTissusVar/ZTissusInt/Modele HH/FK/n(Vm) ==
  note: V
  note: alpha_*(1-n)
  note: beta_n*n
  note: n
  note: n
  Vm : Inport  Port=1  LatchInput=off
  (1-n) : Fcn  Expr=1-u
  Integrator1 : Integrator  InitialCondition=n0
  Product : Product
  Product1 : Product
  Sum1 : Sum  Inputs=+-
  V : Fcn  Expr=u-Vr
  alpha_n : Fcn  Expr=(0.01*(10-u))/(exp((10-u)/10)-1)
  beta_n : Fcn  Expr=0.125*exp(-u/80)
  n : Outport  InitialOutput=0
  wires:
  V/1 -> alpha_n/1, beta_n/1
  alpha_n/1 -> Product/2
  (1-n)/1 -> Product/1
  beta_n/1 -> Product1/1
  Product/1 -> Sum1/1
  Product1/1 -> Sum1/2
  Sum1/1 -> Integrator1/1
  Integrator1/1 -> (1-n)/1, Product1/2, n/1
  Vm/1 -> V/1

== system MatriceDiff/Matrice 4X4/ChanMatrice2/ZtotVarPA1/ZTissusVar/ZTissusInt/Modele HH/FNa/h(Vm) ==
  note: h
  note: h
  note: beta_h*h
  note: alpha_h*(1-h)
  note: V
  Vm : Inport  Port=1  LatchInput=off
  (1-h) : Fcn  Expr=1-u
  Integrator1 : Integrator  InitialCondition=h0
  Product : Product
  Product1 : Product
  Sum1 : Sum  Inputs=+-
  V : Fcn  Expr=u-Vr
  alpha_h : Fcn  Expr=0.07*exp(-u/20)
  beta_h : Fcn  Expr=1/(exp((30-u)/10)+1)
  h : Outport  InitialOutput=0
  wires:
  Vm/1 -> V/1
  Integrator1/1 -> h/1, Product1/2, (1-h)/1
  Sum1/1 -> Integrator1/1
  Product1/1 -> Sum1/2
  Product/1 -> Sum1/1
  beta_h/1 -> Product1/1
  (1-h)/1 -> Product/1
  alpha_h/1 -> Product/2
  V/1 -> beta_h/1, alpha_h/1

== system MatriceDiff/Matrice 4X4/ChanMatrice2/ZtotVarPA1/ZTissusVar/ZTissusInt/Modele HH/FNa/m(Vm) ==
  note: m
  note: m
  note: beta_m*m
  note: alpha_m*(1-m)
  note: V
  Vm : Inport  Port=1  LatchInput=off
  (1-m) : Fcn  Expr=1-u
  Integrator1 : Integrator  InitialCondition=m0
  Product : Product
  Product1 : Product
  Sum1 : Sum  Inputs=+-
  V : Fcn  Expr=u-Vr
  alpha_m : Fcn  Expr=(0.1*(25-u))/(exp((25-u)/10)-1)
  beta_m : Fcn  Expr=4*exp(-u/18)
  n : Outport  InitialOutput=0
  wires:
  Vm/1 -> V/1
  Integrator1/1 -> n/1, Product1/2, (1-m)/1
  Sum1/1 -> Integrator1/1
  Product1/1 -> Sum1/2
  Product/1 -> Sum1/1
  beta_m/1 -> Product1/1
  (1-m)/1 -> Product/1
  alpha_m/1 -> Product/2
  V/1 -> beta_m/1, alpha_m/1

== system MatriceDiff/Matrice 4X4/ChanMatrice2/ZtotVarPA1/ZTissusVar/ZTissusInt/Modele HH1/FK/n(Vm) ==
  note: V
  note: alpha_*(1-n)
  note: beta_n*n
  note: n
  note: n
  Vm : Inport  Port=1  LatchInput=off
  (1-n) : Fcn  Expr=1-u
  Integrator1 : Integrator  InitialCondition=n0
  Product : Product
  Product1 : Product
  Sum1 : Sum  Inputs=+-
  V : Fcn  Expr=u-Vr
  alpha_n : Fcn  Expr=(0.01*(10-u))/(exp((10-u)/10)-1)
  beta_n : Fcn  Expr=0.125*exp(-u/80)
  n : Outport  InitialOutput=0
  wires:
  V/1 -> alpha_n/1, beta_n/1
  alpha_n/1 -> Product/2
  (1-n)/1 -> Product/1
  beta_n/1 -> Product1/1
  Product/1 -> Sum1/1
  Product1/1 -> Sum1/2
  Sum1/1 -> Integrator1/1
  Integrator1/1 -> (1-n)/1, Product1/2, n/1
  Vm/1 -> V/1

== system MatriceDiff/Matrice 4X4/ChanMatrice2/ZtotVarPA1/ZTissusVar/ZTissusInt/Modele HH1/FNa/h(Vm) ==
  note: h
  note: h
  note: beta_h*h
  note: alpha_h*(1-h)
  note: V
  Vm : Inport  Port=1  LatchInput=off
  (1-h) : Fcn  Expr=1-u
  Integrator1 : Integrator  InitialCondition=h0
  Product : Product
  Product1 : Product
  Sum1 : Sum  Inputs=+-
  V : Fcn  Expr=u-Vr
  alpha_h : Fcn  Expr=0.07*exp(-u/20)
  beta_h : Fcn  Expr=1/(exp((30-u)/10)+1)
  h : Outport  InitialOutput=0
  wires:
  Vm/1 -> V/1
  Integrator1/1 -> h/1, Product1/2, (1-h)/1
  Sum1/1 -> Integrator1/1
  Product1/1 -> Sum1/2
  Product/1 -> Sum1/1
  beta_h/1 -> Product1/1
  (1-h)/1 -> Product/1
  alpha_h/1 -> Product/2
  V/1 -> beta_h/1, alpha_h/1

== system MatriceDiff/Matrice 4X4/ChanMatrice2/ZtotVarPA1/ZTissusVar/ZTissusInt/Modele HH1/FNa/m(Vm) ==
  note: m
  note: m
  note: beta_m*m
  note: alpha_m*(1-m)
  note: V
  Vm : Inport  Port=1  LatchInput=off
  (1-m) : Fcn  Expr=1-u
  Integrator1 : Integrator  InitialCondition=m0
  Product : Product
  Product1 : Product
  Sum1 : Sum  Inputs=+-
  V : Fcn  Expr=u-Vr
  alpha_m : Fcn  Expr=(0.1*(25-u))/(exp((25-u)/10)-1)
  beta_m : Fcn  Expr=4*exp(-u/18)
  n : Outport  InitialOutput=0
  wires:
  Vm/1 -> V/1
  Integrator1/1 -> n/1, Product1/2, (1-m)/1
  Sum1/1 -> Integrator1/1
  Product1/1 -> Sum1/2
  Product/1 -> Sum1/1
  beta_m/1 -> Product1/1
  (1-m)/1 -> Product/1
  alpha_m/1 -> Product/2
  V/1 -> beta_m/1, alpha_m/1

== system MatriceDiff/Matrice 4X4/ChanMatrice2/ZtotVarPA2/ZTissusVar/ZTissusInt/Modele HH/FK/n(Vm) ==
  note: V
  note: alpha_*(1-n)
  note: beta_n*n
  note: n
  note: n
  Vm : Inport  Port=1  LatchInput=off
  (1-n) : Fcn  Expr=1-u
  Integrator1 : Integrator  InitialCondition=n0
  Product : Product
  Product1 : Product
  Sum1 : Sum  Inputs=+-
  V : Fcn  Expr=u-Vr
  alpha_n : Fcn  Expr=(0.01*(10-u))/(exp((10-u)/10)-1)
  beta_n : Fcn  Expr=0.125*exp(-u/80)
  n : Outport  InitialOutput=0
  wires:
  V/1 -> alpha_n/1, beta_n/1
  alpha_n/1 -> Product/2
  (1-n)/1 -> Product/1
  beta_n/1 -> Product1/1
  Product/1 -> Sum1/1
  Product1/1 -> Sum1/2
  Sum1/1 -> Integrator1/1
  Integrator1/1 -> (1-n)/1, Product1/2, n/1
  Vm/1 -> V/1

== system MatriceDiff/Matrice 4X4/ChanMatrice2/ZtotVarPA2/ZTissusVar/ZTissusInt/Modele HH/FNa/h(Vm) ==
  note: h
  note: h
  note: beta_h*h
  note: alpha_h*(1-h)
  note: V
  Vm : Inport  Port=1  LatchInput=off
  (1-h) : Fcn  Expr=1-u
  Integrator1 : Integrator  InitialCondition=h0
  Product : Product
  Product1 : Product
  Sum1 : Sum  Inputs=+-
  V : Fcn  Expr=u-Vr
  alpha_h : Fcn  Expr=0.07*exp(-u/20)
  beta_h : Fcn  Expr=1/(exp((30-u)/10)+1)
  h : Outport  InitialOutput=0
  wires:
  Vm/1 -> V/1
  Integrator1/1 -> h/1, Product1/2, (1-h)/1
  Sum1/1 -> Integrator1/1
  Product1/1 -> Sum1/2
  Product/1 -> Sum1/1
  beta_h/1 -> Product1/1
  (1-h)/1 -> Product/1
  alpha_h/1 -> Product/2
  V/1 -> beta_h/1, alpha_h/1

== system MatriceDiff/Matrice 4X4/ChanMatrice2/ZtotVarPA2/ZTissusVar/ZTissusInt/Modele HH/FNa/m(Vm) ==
  note: m
  note: m
  note: beta_m*m
  note: alpha_m*(1-m)
  note: V
  Vm : Inport  Port=1  LatchInput=off
  (1-m) : Fcn  Expr=1-u
  Integrator1 : Integrator  InitialCondition=m0
  Product : Product
  Product1 : Product
  Sum1 : Sum  Inputs=+-
  V : Fcn  Expr=u-Vr
  alpha_m : Fcn  Expr=(0.1*(25-u))/(exp((25-u)/10)-1)
  beta_m : Fcn  Expr=4*exp(-u/18)
  n : Outport  InitialOutput=0
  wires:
  Vm/1 -> V/1
  Integrator1/1 -> n/1, Product1/2, (1-m)/1
  Sum1/1 -> Integrator1/1
  Product1/1 -> Sum1/2
  Product/1 -> Sum1/1
  beta_m/1 -> Product1/1
  (1-m)/1 -> Product/1
  alpha_m/1 -> Product/2
  V/1 -> beta_m/1, alpha_m/1

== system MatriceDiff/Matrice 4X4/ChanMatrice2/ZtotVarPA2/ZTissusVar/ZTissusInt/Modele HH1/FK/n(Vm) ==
  note: V
  note: alpha_*(1-n)
  note: beta_n*n
  note: n
  note: n
  Vm : Inport  Port=1  LatchInput=off
  (1-n) : Fcn  Expr=1-u
  Integrator1 : Integrator  InitialCondition=n0
  Product : Product
  Product1 : Product
  Sum1 : Sum  Inputs=+-
  V : Fcn  Expr=u-Vr
  alpha_n : Fcn  Expr=(0.01*(10-u))/(exp((10-u)/10)-1)
  beta_n : Fcn  Expr=0.125*exp(-u/80)
  n : Outport  InitialOutput=0
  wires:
  V/1 -> alpha_n/1, beta_n/1
  alpha_n/1 -> Product/2
  (1-n)/1 -> Product/1
  beta_n/1 -> Product1/1
  Product/1 -> Sum1/1
  Product1/1 -> Sum1/2
  Sum1/1 -> Integrator1/1
  Integrator1/1 -> (1-n)/1, Product1/2, n/1
  Vm/1 -> V/1

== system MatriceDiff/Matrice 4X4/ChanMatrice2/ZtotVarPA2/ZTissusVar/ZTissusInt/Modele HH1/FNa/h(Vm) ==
  note: h
  note: h
  note: beta_h*h
  note: alpha_h*(1-h)
  note: V
  Vm : Inport  Port=1  LatchInput=off
  (1-h) : Fcn  Expr=1-u
  Integrator1 : Integrator  InitialCondition=h0
  Product : Product
  Product1 : Product
  Sum1 : Sum  Inputs=+-
  V : Fcn  Expr=u-Vr
  alpha_h : Fcn  Expr=0.07*exp(-u/20)
  beta_h : Fcn  Expr=1/(exp((30-u)/10)+1)
  h : Outport  InitialOutput=0
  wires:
  Vm/1 -> V/1
  Integrator1/1 -> h/1, Product1/2, (1-h)/1
  Sum1/1 -> Integrator1/1
  Product1/1 -> Sum1/2
  Product/1 -> Sum1/1
  beta_h/1 -> Product1/1
  (1-h)/1 -> Product/1
  alpha_h/1 -> Product/2
  V/1 -> beta_h/1, alpha_h/1

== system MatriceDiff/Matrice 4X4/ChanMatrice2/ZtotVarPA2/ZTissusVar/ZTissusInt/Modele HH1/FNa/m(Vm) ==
  note: m
  note: m
  note: beta_m*m
  note: alpha_m*(1-m)
  note: V
  Vm : Inport  Port=1  LatchInput=off
  (1-m) : Fcn  Expr=1-u
  Integrator1 : Integrator  InitialCondition=m0
  Product : Product
  Product1 : Product
  Sum1 : Sum  Inputs=+-
  V : Fcn  Expr=u-Vr
  alpha_m : Fcn  Expr=(0.1*(25-u))/(exp((25-u)/10)-1)
  beta_m : Fcn  Expr=4*exp(-u/18)
  n : Outport  InitialOutput=0
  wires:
  Vm/1 -> V/1
  Integrator1/1 -> n/1, Product1/2, (1-m)/1
  Sum1/1 -> Integrator1/1
  Product1/1 -> Sum1/2
  Product/1 -> Sum1/1
  beta_m/1 -> Product1/1
  (1-m)/1 -> Product/1
  alpha_m/1 -> Product/2
  V/1 -> beta_m/1, alpha_m/1

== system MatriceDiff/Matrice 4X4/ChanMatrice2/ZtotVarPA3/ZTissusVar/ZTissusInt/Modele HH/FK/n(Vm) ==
  note: V
  note: alpha_*(1-n)
  note: beta_n*n
  note: n
  note: n
  Vm : Inport  Port=1  LatchInput=off
  (1-n) : Fcn  Expr=1-u
  Integrator1 : Integrator  InitialCondition=n0
  Product : Product
  Product1 : Product
  Sum1 : Sum  Inputs=+-
  V : Fcn  Expr=u-Vr
  alpha_n : Fcn  Expr=(0.01*(10-u))/(exp((10-u)/10)-1)
  beta_n : Fcn  Expr=0.125*exp(-u/80)
  n : Outport  InitialOutput=0
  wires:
  V/1 -> alpha_n/1, beta_n/1
  alpha_n/1 -> Product/2
  (1-n)/1 -> Product/1
  beta_n/1 -> Product1/1
  Product/1 -> Sum1/1
  Product1/1 -> Sum1/2
  Sum1/1 -> Integrator1/1
  Integrator1/1 -> (1-n)/1, Product1/2, n/1
  Vm/1 -> V/1

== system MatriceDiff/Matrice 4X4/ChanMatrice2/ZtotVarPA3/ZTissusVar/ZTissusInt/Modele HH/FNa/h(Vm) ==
  note: h
  note: h
  note: beta_h*h
  note: alpha_h*(1-h)
  note: V
  Vm : Inport  Port=1  LatchInput=off
  (1-h) : Fcn  Expr=1-u
  Integrator1 : Integrator  InitialCondition=h0
  Product : Product
  Product1 : Product
  Sum1 : Sum  Inputs=+-
  V : Fcn  Expr=u-Vr
  alpha_h : Fcn  Expr=0.07*exp(-u/20)
  beta_h : Fcn  Expr=1/(exp((30-u)/10)+1)
  h : Outport  InitialOutput=0
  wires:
  Vm/1 -> V/1
  Integrator1/1 -> h/1, Product1/2, (1-h)/1
  Sum1/1 -> Integrator1/1
  Product1/1 -> Sum1/2
  Product/1 -> Sum1/1
  beta_h/1 -> Product1/1
  (1-h)/1 -> Product/1
  alpha_h/1 -> Product/2
  V/1 -> beta_h/1, alpha_h/1

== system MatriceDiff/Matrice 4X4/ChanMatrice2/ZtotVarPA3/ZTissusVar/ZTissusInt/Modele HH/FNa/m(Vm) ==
  note: m
  note: m
  note: beta_m*m
  note: alpha_m*(1-m)
  note: V
  Vm : Inport  Port=1  LatchInput=off
  (1-m) : Fcn  Expr=1-u
  Integrator1 : Integrator  InitialCondition=m0
  Product : Product
  Product1 : Product
  Sum1 : Sum  Inputs=+-
  V : Fcn  Expr=u-Vr
  alpha_m : Fcn  Expr=(0.1*(25-u))/(exp((25-u)/10)-1)
  beta_m : Fcn  Expr=4*exp(-u/18)
  n : Outport  InitialOutput=0
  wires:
  Vm/1 -> V/1
  Integrator1/1 -> n/1, Product1/2, (1-m)/1
  Sum1/1 -> Integrator1/1
  Product1/1 -> Sum1/2
  Product/1 -> Sum1/1
  beta_m/1 -> Product1/1
  (1-m)/1 -> Product/1
  alpha_m/1 -> Product/2
  V/1 -> beta_m/1, alpha_m/1

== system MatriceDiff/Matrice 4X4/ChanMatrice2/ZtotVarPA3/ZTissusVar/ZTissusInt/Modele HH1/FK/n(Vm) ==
  note: V
  note: alpha_*(1-n)
  note: beta_n*n
  note: n
  note: n
  Vm : Inport  Port=1  LatchInput=off
  (1-n) : Fcn  Expr=1-u
  Integrator1 : Integrator  InitialCondition=n0
  Product : Product
  Product1 : Product
  Sum1 : Sum  Inputs=+-
  V : Fcn  Expr=u-Vr
  alpha_n : Fcn  Expr=(0.01*(10-u))/(exp((10-u)/10)-1)
  beta_n : Fcn  Expr=0.125*exp(-u/80)
  n : Outport  InitialOutput=0
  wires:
  V/1 -> alpha_n/1, beta_n/1
  alpha_n/1 -> Product/2
  (1-n)/1 -> Product/1
  beta_n/1 -> Product1/1
  Product/1 -> Sum1/1
  Product1/1 -> Sum1/2
  Sum1/1 -> Integrator1/1
  Integrator1/1 -> (1-n)/1, Product1/2, n/1
  Vm/1 -> V/1

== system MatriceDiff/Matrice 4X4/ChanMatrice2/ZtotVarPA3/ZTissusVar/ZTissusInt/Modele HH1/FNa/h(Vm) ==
  note: h
  note: h
  note: beta_h*h
  note: alpha_h*(1-h)
  note: V
  Vm : Inport  Port=1  LatchInput=off
  (1-h) : Fcn  Expr=1-u
  Integrator1 : Integrator  InitialCondition=h0
  Product : Product
  Product1 : Product
  Sum1 : Sum  Inputs=+-
  V : Fcn  Expr=u-Vr
  alpha_h : Fcn  Expr=0.07*exp(-u/20)
  beta_h : Fcn  Expr=1/(exp((30-u)/10)+1)
  h : Outport  InitialOutput=0
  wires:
  Vm/1 -> V/1
  Integrator1/1 -> h/1, Product1/2, (1-h)/1
  Sum1/1 -> Integrator1/1
  Product1/1 -> Sum1/2
  Product/1 -> Sum1/1
  beta_h/1 -> Product1/1
  (1-h)/1 -> Product/1
  alpha_h/1 -> Product/2
  V/1 -> beta_h/1, alpha_h/1

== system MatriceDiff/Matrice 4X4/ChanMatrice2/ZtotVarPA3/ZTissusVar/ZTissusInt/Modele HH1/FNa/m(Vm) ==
  note: m
  note: m
  note: beta_m*m
  note: alpha_m*(1-m)
  note: V
  Vm : Inport  Port=1  LatchInput=off
  (1-m) : Fcn  Expr=1-u
  Integrator1 : Integrator  InitialCondition=m0
  Product : Product
  Product1 : Product
  Sum1 : Sum  Inputs=+-
  V : Fcn  Expr=u-Vr
  alpha_m : Fcn  Expr=(0.1*(25-u))/(exp((25-u)/10)-1)
  beta_m : Fcn  Expr=4*exp(-u/18)
  n : Outport  InitialOutput=0
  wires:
  Vm/1 -> V/1
  Integrator1/1 -> n/1, Product1/2, (1-m)/1
  Sum1/1 -> Integrator1/1
  Product1/1 -> Sum1/2
  Product/1 -> Sum1/1
  beta_m/1 -> Product1/1
  (1-m)/1 -> Product/1
  alpha_m/1 -> Product/2
  V/1 -> beta_m/1, alpha_m/1

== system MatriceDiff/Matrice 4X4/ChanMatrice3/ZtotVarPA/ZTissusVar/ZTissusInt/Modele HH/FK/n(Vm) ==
  note: V
  note: alpha_*(1-n)
  note: beta_n*n
  note: n
  note: n
  Vm : Inport  Port=1  LatchInput=off
  (1-n) : Fcn  Expr=1-u
  Integrator1 : Integrator  InitialCondition=n0
  Product : Product
  Product1 : Product
  Sum1 : Sum  Inputs=+-
  V : Fcn  Expr=u-Vr
  alpha_n : Fcn  Expr=(0.01*(10-u))/(exp((10-u)/10)-1)
  beta_n : Fcn  Expr=0.125*exp(-u/80)
  n : Outport  InitialOutput=0
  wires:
  V/1 -> alpha_n/1, beta_n/1
  alpha_n/1 -> Product/2
  (1-n)/1 -> Product/1
  beta_n/1 -> Product1/1
  Product/1 -> Sum1/1
  Product1/1 -> Sum1/2
  Sum1/1 -> Integrator1/1
  Integrator1/1 -> (1-n)/1, Product1/2, n/1
  Vm/1 -> V/1

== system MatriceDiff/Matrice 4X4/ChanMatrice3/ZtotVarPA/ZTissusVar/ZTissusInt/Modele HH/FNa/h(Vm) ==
  note: h
  note: h
  note: beta_h*h
  note: alpha_h*(1-h)
  note: V
  Vm : Inport  Port=1  LatchInput=off
  (1-h) : Fcn  Expr=1-u
  Integrator1 : Integrator  InitialCondition=h0
  Product : Product
  Product1 : Product
  Sum1 : Sum  Inputs=+-
  V : Fcn  Expr=u-Vr
  alpha_h : Fcn  Expr=0.07*exp(-u/20)
  beta_h : Fcn  Expr=1/(exp((30-u)/10)+1)
  h : Outport  InitialOutput=0
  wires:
  Vm/1 -> V/1
  Integrator1/1 -> h/1, Product1/2, (1-h)/1
  Sum1/1 -> Integrator1/1
  Product1/1 -> Sum1/2
  Product/1 -> Sum1/1
  beta_h/1 -> Product1/1
  (1-h)/1 -> Product/1
  alpha_h/1 -> Product/2
  V/1 -> beta_h/1, alpha_h/1

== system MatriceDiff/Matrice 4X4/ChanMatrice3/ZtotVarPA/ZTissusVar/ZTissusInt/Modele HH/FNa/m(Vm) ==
  note: m
  note: m
  note: beta_m*m
  note: alpha_m*(1-m)
  note: V
  Vm : Inport  Port=1  LatchInput=off
  (1-m) : Fcn  Expr=1-u
  Integrator1 : Integrator  InitialCondition=m0
  Product : Product
  Product1 : Product
  Sum1 : Sum  Inputs=+-
  V : Fcn  Expr=u-Vr
  alpha_m : Fcn  Expr=(0.1*(25-u))/(exp((25-u)/10)-1)
  beta_m : Fcn  Expr=4*exp(-u/18)
  n : Outport  InitialOutput=0
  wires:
  Vm/1 -> V/1
  Integrator1/1 -> n/1, Product1/2, (1-m)/1
  Sum1/1 -> Integrator1/1
  Product1/1 -> Sum1/2
  Product/1 -> Sum1/1
  beta_m/1 -> Product1/1
  (1-m)/1 -> Product/1
  alpha_m/1 -> Product/2
  V/1 -> beta_m/1, alpha_m/1

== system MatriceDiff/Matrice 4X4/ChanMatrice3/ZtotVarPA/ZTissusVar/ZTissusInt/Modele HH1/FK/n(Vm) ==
  note: V
  note: alpha_*(1-n)
  note: beta_n*n
  note: n
  note: n
  Vm : Inport  Port=1  LatchInput=off
  (1-n) : Fcn  Expr=1-u
  Integrator1 : Integrator  InitialCondition=n0
  Product : Product
  Product1 : Product
  Sum1 : Sum  Inputs=+-
  V : Fcn  Expr=u-Vr
  alpha_n : Fcn  Expr=(0.01*(10-u))/(exp((10-u)/10)-1)
  beta_n : Fcn  Expr=0.125*exp(-u/80)
  n : Outport  InitialOutput=0
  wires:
  V/1 -> alpha_n/1, beta_n/1
  alpha_n/1 -> Product/2
  (1-n)/1 -> Product/1
  beta_n/1 -> Product1/1
  Product/1 -> Sum1/1
  Product1/1 -> Sum1/2
  Sum1/1 -> Integrator1/1
  Integrator1/1 -> (1-n)/1, Product1/2, n/1
  Vm/1 -> V/1

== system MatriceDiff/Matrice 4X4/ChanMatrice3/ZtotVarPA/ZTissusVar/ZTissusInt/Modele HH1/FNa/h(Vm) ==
  note: h
  note: h
  note: beta_h*h
  note: alpha_h*(1-h)
  note: V
  Vm : Inport  Port=1  LatchInput=off
  (1-h) : Fcn  Expr=1-u
  Integrator1 : Integrator  InitialCondition=h0
  Product : Product
  Product1 : Product
  Sum1 : Sum  Inputs=+-
  V : Fcn  Expr=u-Vr
  alpha_h : Fcn  Expr=0.07*exp(-u/20)
  beta_h : Fcn  Expr=1/(exp((30-u)/10)+1)
  h : Outport  InitialOutput=0
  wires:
  Vm/1 -> V/1
  Integrator1/1 -> h/1, Product1/2, (1-h)/1
  Sum1/1 -> Integrator1/1
  Product1/1 -> Sum1/2
  Product/1 -> Sum1/1
  beta_h/1 -> Product1/1
  (1-h)/1 -> Product/1
  alpha_h/1 -> Product/2
  V/1 -> beta_h/1, alpha_h/1

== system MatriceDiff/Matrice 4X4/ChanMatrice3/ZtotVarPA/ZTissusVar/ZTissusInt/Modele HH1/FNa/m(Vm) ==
  note: m
  note: m
  note: beta_m*m
  note: alpha_m*(1-m)
  note: V
  Vm : Inport  Port=1  LatchInput=off
  (1-m) : Fcn  Expr=1-u
  Integrator1 : Integrator  InitialCondition=m0
  Product : Product
  Product1 : Product
  Sum1 : Sum  Inputs=+-
  V : Fcn  Expr=u-Vr
  alpha_m : Fcn  Expr=(0.1*(25-u))/(exp((25-u)/10)-1)
  beta_m : Fcn  Expr=4*exp(-u/18)
  n : Outport  InitialOutput=0
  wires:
  Vm/1 -> V/1
  Integrator1/1 -> n/1, Product1/2, (1-m)/1
  Sum1/1 -> Integrator1/1
  Product1/1 -> Sum1/2
  Product/1 -> Sum1/1
  beta_m/1 -> Product1/1
  (1-m)/1 -> Product/1
  alpha_m/1 -> Product/2
  V/1 -> beta_m/1, alpha_m/1

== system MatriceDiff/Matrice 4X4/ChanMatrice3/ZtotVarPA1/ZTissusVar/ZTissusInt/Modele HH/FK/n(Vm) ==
  note: V
  note: alpha_*(1-n)
  note: beta_n*n
  note: n
  note: n
  Vm : Inport  Port=1  LatchInput=off
  (1-n) : Fcn  Expr=1-u
  Integrator1 : Integrator  InitialCondition=n0
  Product : Product
  Product1 : Product
  Sum1 : Sum  Inputs=+-
  V : Fcn  Expr=u-Vr
  alpha_n : Fcn  Expr=(0.01*(10-u))/(exp((10-u)/10)-1)
  beta_n : Fcn  Expr=0.125*exp(-u/80)
  n : Outport  InitialOutput=0
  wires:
  V/1 -> alpha_n/1, beta_n/1
  alpha_n/1 -> Product/2
  (1-n)/1 -> Product/1
  beta_n/1 -> Product1/1
  Product/1 -> Sum1/1
  Product1/1 -> Sum1/2
  Sum1/1 -> Integrator1/1
  Integrator1/1 -> (1-n)/1, Product1/2, n/1
  Vm/1 -> V/1

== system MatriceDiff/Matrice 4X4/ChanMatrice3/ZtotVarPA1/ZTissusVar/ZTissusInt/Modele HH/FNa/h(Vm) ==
  note: h
  note: h
  note: beta_h*h
  note: alpha_h*(1-h)
  note: V
  Vm : Inport  Port=1  LatchInput=off
  (1-h) : Fcn  Expr=1-u
  Integrator1 : Integrator  InitialCondition=h0
  Product : Product
  Product1 : Product
  Sum1 : Sum  Inputs=+-
  V : Fcn  Expr=u-Vr
  alpha_h : Fcn  Expr=0.07*exp(-u/20)
  beta_h : Fcn  Expr=1/(exp((30-u)/10)+1)
  h : Outport  InitialOutput=0
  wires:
  Vm/1 -> V/1
  Integrator1/1 -> h/1, Product1/2, (1-h)/1
  Sum1/1 -> Integrator1/1
  Product1/1 -> Sum1/2
  Product/1 -> Sum1/1
  beta_h/1 -> Product1/1
  (1-h)/1 -> Product/1
  alpha_h/1 -> Product/2
  V/1 -> beta_h/1, alpha_h/1

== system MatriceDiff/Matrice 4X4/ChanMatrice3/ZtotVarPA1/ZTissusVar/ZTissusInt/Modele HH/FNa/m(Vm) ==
  note: m
  note: m
  note: beta_m*m
  note: alpha_m*(1-m)
  note: V
  Vm : Inport  Port=1  LatchInput=off
  (1-m) : Fcn  Expr=1-u
  Integrator1 : Integrator  InitialCondition=m0
  Product : Product
  Product1 : Product
  Sum1 : Sum  Inputs=+-
  V : Fcn  Expr=u-Vr
  alpha_m : Fcn  Expr=(0.1*(25-u))/(exp((25-u)/10)-1)
  beta_m : Fcn  Expr=4*exp(-u/18)
  n : Outport  InitialOutput=0
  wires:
  Vm/1 -> V/1
  Integrator1/1 -> n/1, Product1/2, (1-m)/1
  Sum1/1 -> Integrator1/1
  Product1/1 -> Sum1/2
  Product/1 -> Sum1/1
  beta_m/1 -> Product1/1
  (1-m)/1 -> Product/1
  alpha_m/1 -> Product/2
  V/1 -> beta_m/1, alpha_m/1
